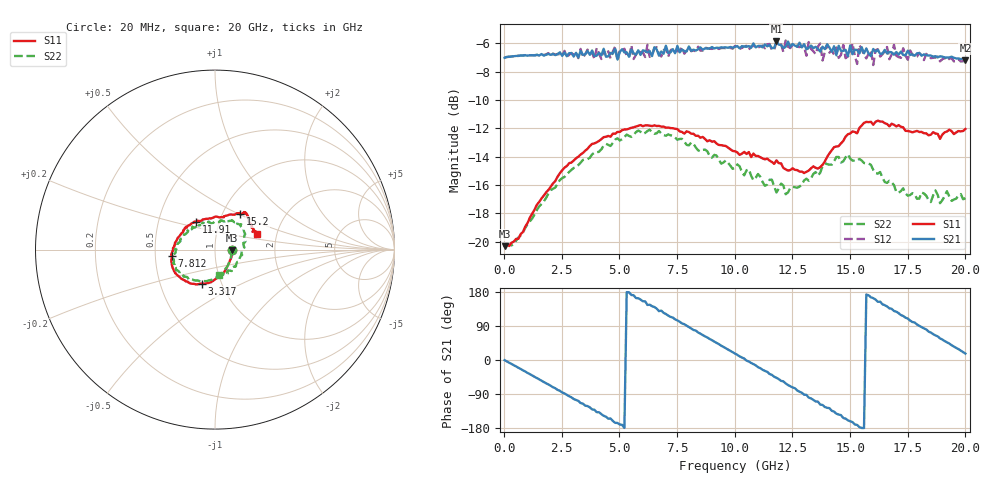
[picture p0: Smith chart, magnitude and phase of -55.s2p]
!Agilent Technologies,N5230A,US43500223,A.07.50.48
!Agilent N5230A: A.07.50.48
!Date: Thursday, September 17, 2015 17:10:23
!Correction: S11(Full 2 Port(1,2))
!S21(Full 2 Port(1,2))
!S12(Full 2 Port(1,2))
!S22(Full 2 Port(1,2))
!S2P File: Measurements: S11, S21, S12, S22:
# Hz S  dB  R 50
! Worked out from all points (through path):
!   201 points, 20 MHz to 20 GHz, reference 50 ohm
!   highest |S21| = -5.86 dB at 11.81 GHz (marker M1); lowest = -7.2 dB at 20 GHz (marker M2)
!   group delay of S21, straight-line fit = 97.6 ps
!   lowest |S11| = -20.3 dB at 20 MHz (marker M3), VSWR 1.21, Z = 60.7 - j0.401 ohm
!   |S11| at or under -10 dB: start of sweep to end of sweep
!   |S22| runs from -20.3 to -12.1 dB; largest |S21 - S12| = 0.067
!   S11 on the Smith chart (normalised r, x): 20 MHz: 1.21, -0.01; 3.317 GHz: 0.81, -0.32; 7.812 GHz: 0.61, -0.04; 11.91 GHz: 0.77, +0.25; 15.2 GHz: 1.21, +0.51; 20 GHz: 1.58, +0.29
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2e7  -20.32 -1.9  -7.01 -0.5  -6.98 -0.7  -20.26 -1.6
1.9181e9  -16.35 -81.0  -6.73 -64.4  -6.68 -64.5  -16.60 -81.0
3.3167e9  -13.85 -110.4  -6.53 -113.6  -6.38 -113.2  -14.42 -112.1
3.4166e9  -13.73 -112.6  -6.80 -115.4  -7.00 -117.4  -14.23 -113.1
4.8152e9  -12.38 -134.7  -6.38 -165.9  -6.22 -165.0  -12.79 -138.7
5.5145e9  -11.96 -144.4  -6.43 171.6  -6.14 172.1  -12.60 -148.3
6.7133e9  -11.82 -158.4  -6.86 128.9  -6.76 128.6  -12.18 -161.9
7.8122e9  -12.37 -172.0  -6.55 94.5  -6.72 93.3  -12.92 -174.2
8.7113e9  -12.75 176.7  -6.34 62.3  -6.29 63.2  -13.50 171.6
1.001e10  -13.61 155.1  -6.24 16.9  -6.18 16.8  -14.79 144.8
1.08092e10  -13.78 141.4  -6.00 -10.9  -6.12 -11.0  -15.66 131.5
1.18082e10  -14.26 126.6  -5.86 -46.9  -5.91 -46.5  -16.53 106.3
1.19081e10  -14.46 124.2  -6.09 -50.5  -6.10 -53.8  -16.24 104.7
1.28072e10  -15.05 104.1  -5.94 -83.8  -6.26 -82.4  -16.11 80.6
1.34066e10  -14.68 88.0  -6.33 -105.2  -6.55 -108.7  -15.22 68.6
1.4006e10  -14.02 71.6  -6.06 -126.2  -6.07 -124.1  -14.53 59.7
1.52048e10  -12.25 54.5  -6.44 -170.1  -6.85 -170.7  -14.30 37.3
1.61039e10  -11.54 49.6  -6.58 159.7  -6.47 161.0  -15.16 20.8
1.67033e10  -11.86 46.3  -6.60 136.4  -7.12 137.1  -15.70 4.0
1.73027e10  -11.93 41.4  -6.81 116.1  -6.34 115.3  -16.23 -11.1
1.83017e10  -12.35 31.7  -6.83 80.7  -6.74 80.5  -16.75 -40.0
2e10  -12.04 19.8  -7.18 16.9  -7.22 17.7  -16.93 -81.8
